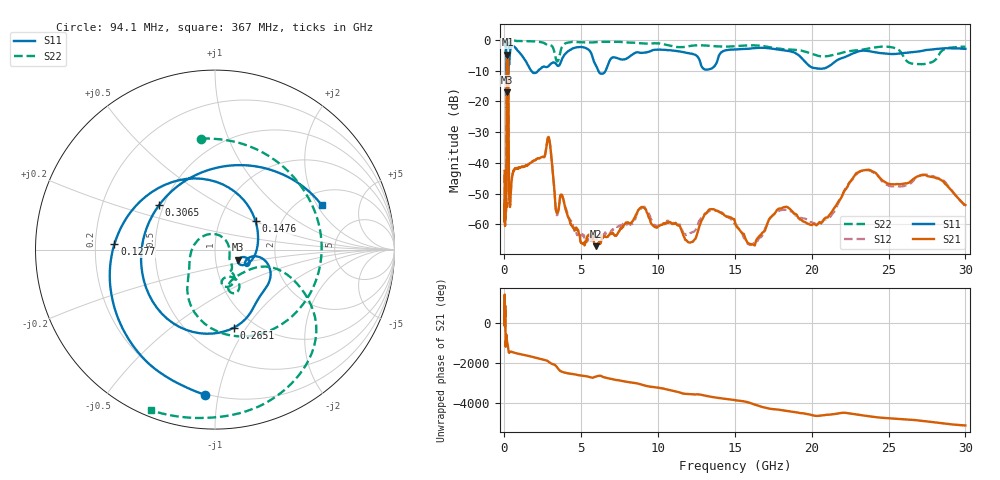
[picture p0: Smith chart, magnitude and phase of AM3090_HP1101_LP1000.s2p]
! Date/Time: Thu, Feb 28, 2019 2:08 PM
! Network Analyzer: Agilent Technologies E8364B Rev: A.07.50.67
! Sweep from 0.010 to 30.000 GHz, 1601 Points, Sweep Type: LOG
! Power Supply: 5.022 V, 0.002 A
# Hz S DB R 50
!freq MagS11 AngS11 MagS21 AngS21 MagS12 AngS12 MagS22 AngS22
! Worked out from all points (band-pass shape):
!   1601 points, 10 MHz to 30 GHz, reference 50 ohm
!   highest |S21| = -4.78 dB at 191.5 MHz (marker M1); lowest = -67.2 dB at 5.959 GHz (marker M2)
!   |S21| within 3 dB of the highest: 151.7 MHz to 244.8 MHz (93.11 MHz wide, 47 % of centre)
!   lowest |S11| = -17.0 dB at 173.3 MHz (marker M3), VSWR 1.33, Z = 64.3 - j7.38 ohm
!   |S11| at or under -10 dB: 144.3 MHz to 227.1 MHz (82.8 MHz wide, 44.6 % of centre); 1.744 GHz to 2.192 GHz (447.4 MHz wide, 22.7 % of centre); 6.109 GHz to 6.584 GHz (474.2 MHz wide, 7.47 % of centre)
!   |S22| runs from -22.1 to -0.1 dB; largest |S21 - S12| = 0.012
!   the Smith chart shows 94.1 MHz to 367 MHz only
!   S11 on the Smith chart (normalised r, x): 94.1 MHz: 0.19, -0.92; 127.7 MHz: 0.28, +0.02; 147.6 MHz: 1.48, +0.51; 265.1 MHz: 0.81, -0.88; 306.5 MHz: 0.47, +0.28; 367 MHz: 2.58, +2.19
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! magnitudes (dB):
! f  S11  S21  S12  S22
! 10 MHz  -0.3  -42.6  -46.7  -0.6
! 38.04 MHz  -0.4  -58.6  -56.8  -1.3
! 94.1 MHz  -1.8  -54.1  -53.6  -4.1
! 116.7 MHz  -3.5  -53.5  -54.6  -4.5
! 127.7 MHz  -5.0  -38.6  -38.1  -5.0
! 144.7 MHz  -10.2  -11.9  -11.8  -19.9
! 147.6 MHz  -11.2  -9.7  -9.6  -21.7
! 173.3 MHz  -17.0  -5.1  -5.0  -15.7
! 191.5 MHz  -13.7  -4.8  -4.8  -13.2
! 243.5 MHz  -8.9  -7.6  -7.5  -14.2
! 265.1 MHz  -7.0  -18.9  -18.9  -7.4
! 306.5 MHz  -8.0  -49.9  -51.2  -0.8
! 367 MHz  -3.8  -54.1  -53.3  -0.3
! 550.5 MHz  -2.0  -43.4  -43.3  -0.2
! 2.084 GHz  -10.6  -38.8  -38.8  -0.5
! 2.884 GHz  -8.4  -31.7  -31.7  -1.8
! 3.419 GHz  -8.2  -56.3  -57.0  -7.0
! 5.959 GHz  -8.4  -67.2  -64.2  -0.7
! 7.926 GHz  -6.1  -59.4  -60.3  -0.8
! 16.21 GHz  -2.7  -66.7  -66.5  -1.7
! 23.48 GHz  -3.5  -42.4  -42.5  -3.0
! 30 GHz  -2.9  -53.7  -54.1  -2.2
